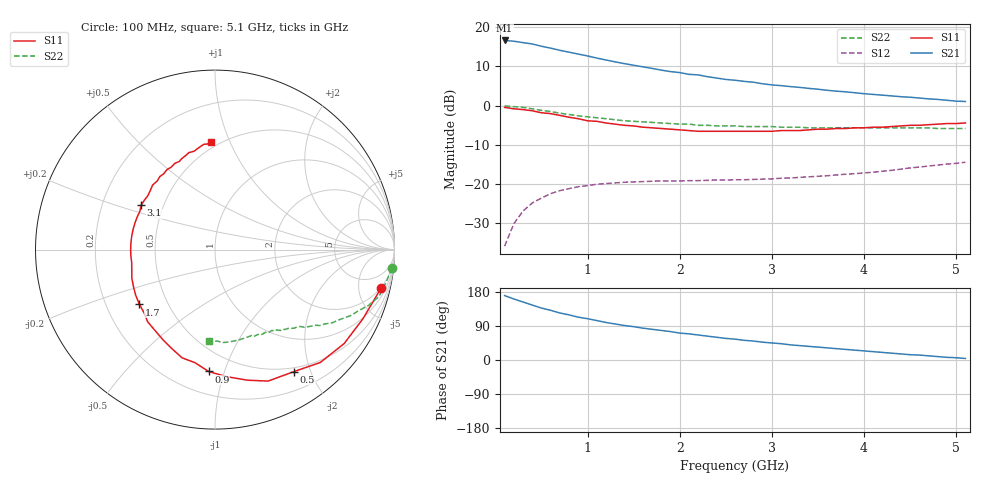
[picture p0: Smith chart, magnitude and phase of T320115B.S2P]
!AT-32011
!S and NOISE PARAMETERS at Vce=5  V  Ic=2mA.  LAST UPDATED 01-05-95
# ghz s ma r 50
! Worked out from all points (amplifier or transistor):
!   51 points, 100 MHz to 5.1 GHz, reference 50 ohm
!   highest |S21| = 16.7 dB at 100 MHz (marker M1)
!   |S21| within 3 dB of that: start of sweep to 802.1 MHz
!   unconditionally stable (mu >= 1): 2.415 GHz to 5.088 GHz
!   at 900 MHz: K = 0.39, MSG = 16.9 dB, |S12| = -20.7 dB
!   at 2.6 GHz: K = 1.03, MAG = 11.6 dB, |S12| = -18.9 dB
!   at 5.1 GHz: K = 1.00, MSG = 7.8 dB, |S12| = -14.5 dB
!   lowest NFmin = 0.52 dB at 500 MHz
!   S11 on the Smith chart (normalised r, x): 100 MHz: 1.90, -8.35; 500 MHz: 0.44, -1.76; 900 MHz: 0.35, -0.89; 1.7 GHz: 0.35, -0.29; 3.1 GHz: 0.37, +0.24; 5.1 GHz: 0.46, +0.86
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0.1  0.95 -13.0  6.8 170.0  0.016 82.0  0.99 -6.0
0.2  0.91 -25.0  6.65 161.0  0.031 75.0  0.97 -11.0
0.3  0.89 -36.0  6.38 153.0  0.045 69.0  0.95 -16.0
0.4  0.86 -47.0  6.13 145.0  0.057 63.0  0.91 -20.0
0.5  0.81 -57.0  5.74 137.0  0.066 58.0  0.87 -23.0
0.7  0.75 -76.0  5.09 124.0  0.082 49.0  0.8 -29.0
0.9  0.68 -93.0  4.55 113.0  0.092 43.0  0.74 -34.0
1  0.64 -100.0  4.31 109.0  0.095 40.0  0.72 -36.0
1.2  0.6 -114.0  3.83 99.0  0.101 36.0  0.68 -39.0
1.3  0.58 -120.0  3.62 95.0  0.103 34.0  0.66 -41.0
1.4  0.56 -127.0  3.44 91.0  0.105 33.0  0.64 -42.0
1.6  0.53 -138.0  3.13 84.0  0.107 31.0  0.62 -45.0
1.7  0.52 -144.0  2.99 81.0  0.108 30.0  0.61 -46.0
1.8  0.51 -150.0  2.84 78.0  0.109 29.0  0.6 -47.0
2  0.49 -161.0  2.64 71.0  0.109 28.0  0.58 -50.0
2.5  0.47 175.0  2.16 57.0  0.112 28.0  0.55 -56.0
2.6  0.47 170.0  2.11 55.0  0.113 29.0  0.55 -57.0
2.9  0.47 157.0  1.9 47.0  0.115 30.0  0.54 -61.0
3.1  0.48 149.0  1.8 43.0  0.118 31.0  0.53 -63.0
3.5  0.5 134.0  1.62 34.0  0.125 34.0  0.52 -68.0
4.3  0.54 110.0  1.33 18.0  0.149 39.0  0.52 -79.0
5.1  0.6 92.0  1.13 4.0  0.189 38.0  0.51 -94.0
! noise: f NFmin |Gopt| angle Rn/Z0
0.5  0.52  0.73  20  0.34
0.9  0.75  0.63  49  0.28
1.8  1.26  0.44  111  0.16
2.4  1.6  0.45  153  0.09
